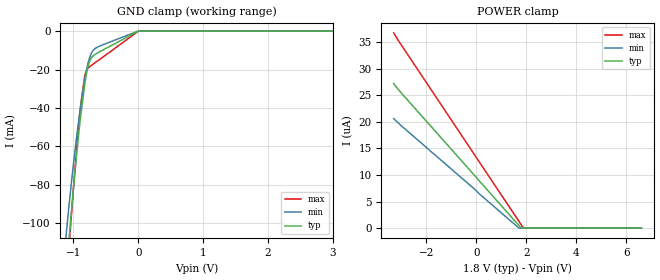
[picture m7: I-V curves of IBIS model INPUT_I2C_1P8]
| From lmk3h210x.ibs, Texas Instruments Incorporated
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[Model]   INPUT_I2C_1P8
Model_type   Input
Vinl = 0.54
Vinh = 1.26
|   typ   min   max
C_comp   0.7pF   0.5pF   0.9pF
[Voltage Range]   1.8   1.71   1.89
[Temperature Range]   45   125   -40
[Power Clamp Reference]   1.8   1.71   1.89
[GND Clamp Reference]   0   0   0
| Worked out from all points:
|   GND clamp passes 1 mA (typ) near -0.06 V on its own axis
[GND Clamp]
|   Voltage   I(typ)   I(min)   I(max)
-3.3V     -1.111A    -994.6mA   -1.235A
-1.181V   -155mA     -130.2mA   -166mA
-1.073V   -110.3mA   -92.21mA   -114.6mA
-1.063V   -106.3mA   -88.93mA   -110.1mA
-1.013V   -87.04mA   -73.2mA    -87.67mA
-943.8mV  -61.84mA   -53.24mA   -58.26mA
-894.3mV  -45.89mA   -40.53mA   -40.04mA
-815.1mV  -25.46mA   -23.28mA   -22mA
-755.7mV  -16.24mA   -14.37mA   -18.73mA
-676.5mV  -12.35mA   -9.42mA    -16.7mA
-3.3mV    -59.89uA   -42.63uA   -82.85uA
6.6V      0A         0A         0A
[POWER Clamp]
|   Voltage   I(typ)   I(min)   I(max)
-3.3V     27.2uA     20.61uA    36.74uA
-2.944V   25.17uA    19.06uA    34.1uA
1.709V    481.2nA    1.046nA    1.274uA
1.798V    7.59nA     0A         645.3nA
1.888V    0A         0A         16.9nA
6.6V      0A         0A         0A
